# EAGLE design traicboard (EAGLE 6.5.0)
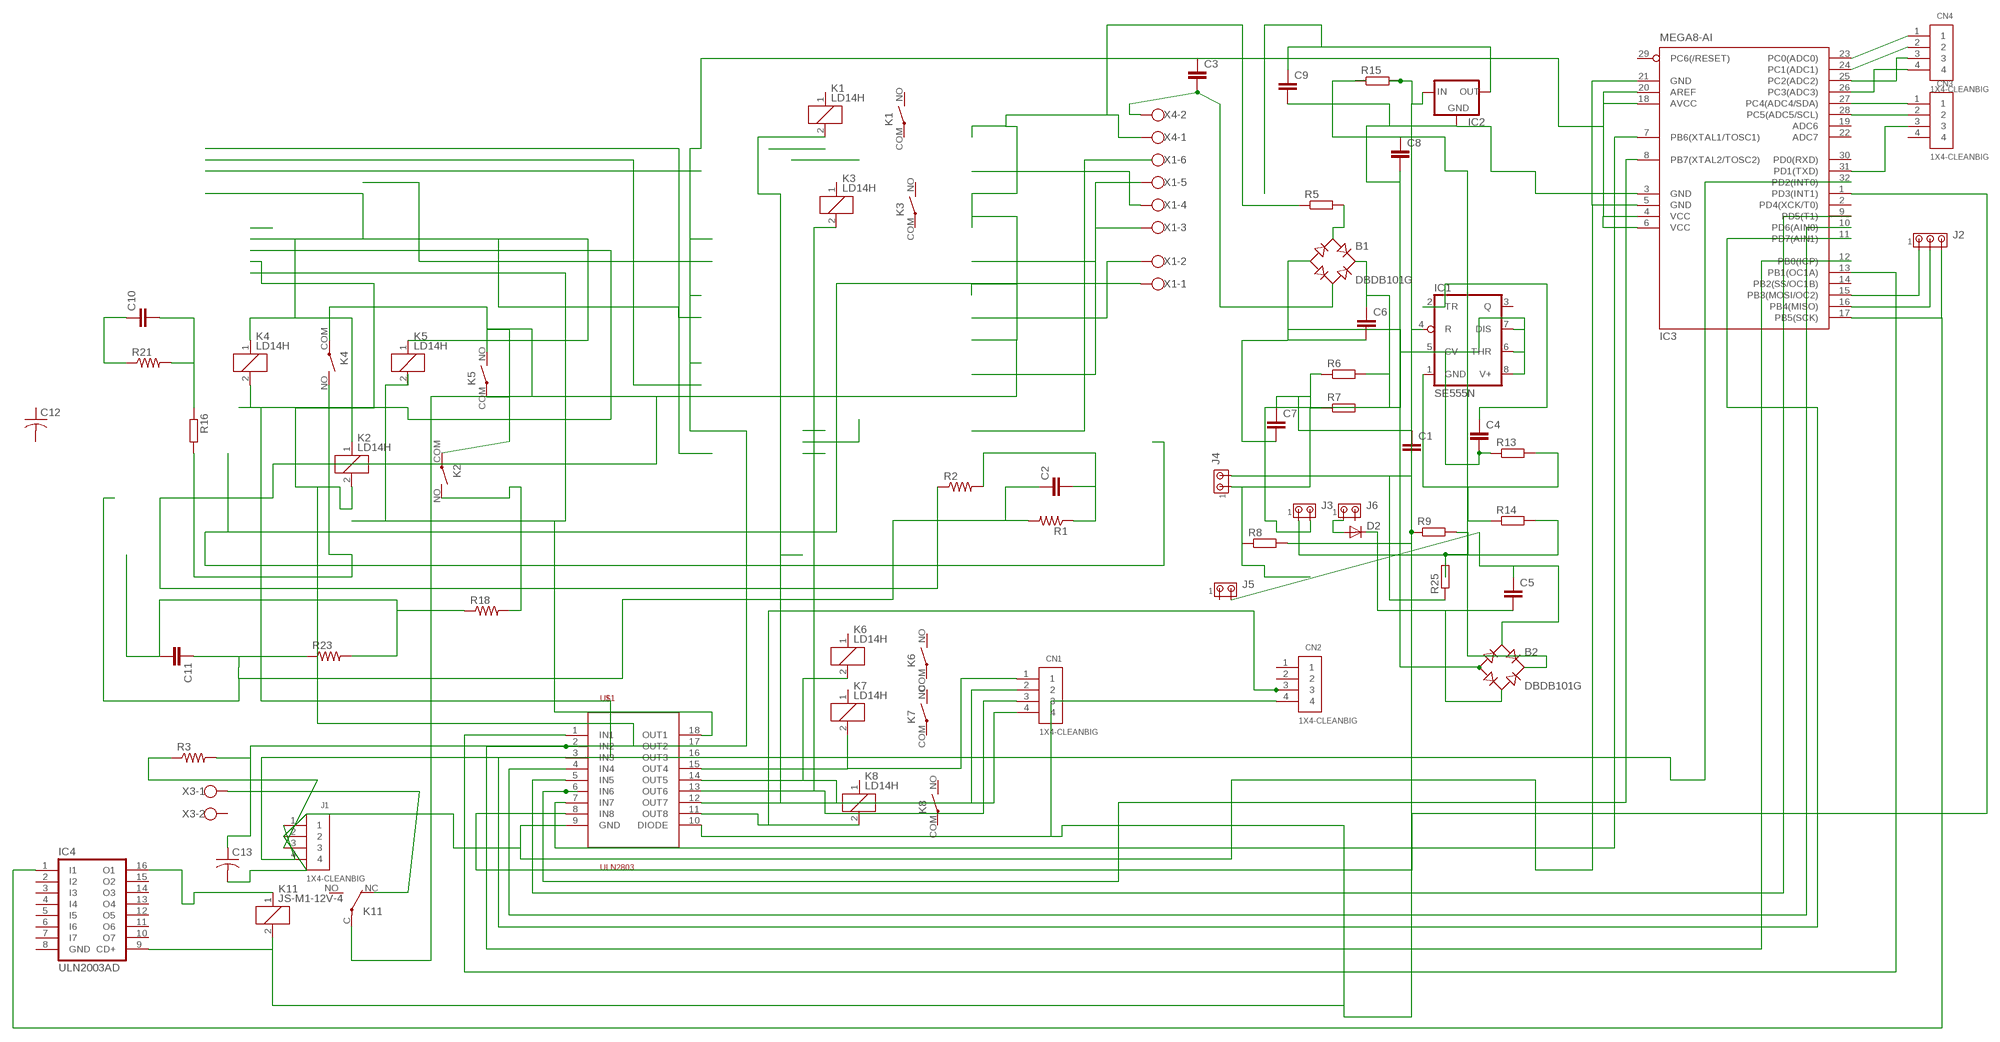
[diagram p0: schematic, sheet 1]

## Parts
B1  DBDB101G  [DB]
B2  DBDB101G  [DB]
C1  C5/2.5  [C5B2.5]
C2  C27/9  [C27.5B9]
C3  C-EU075-032X103  [C075-032X103]
C4  C-EU025-024X044  [C025-024X044]
C5  C-EU025-024X044  [C025-024X044]
C6  C5/2.5  [C5B2.5]
C7  C5/2.5  [C5B2.5]
C8  C-EU025-024X044  [C025-024X044]
C9  C-EU025-024X044  [C025-024X044]
C10  C27/9  [C27.5B9]
C11  C27/9  [C27.5B9]
C12  C-US025-024X044  [C025-024X044]
C13  C-US025-024X044  [C025-024X044]
CN1  1X4-CLEANBIG  [1X04-CLEANBIG]
CN2  1X4-CLEANBIG  [1X04-CLEANBIG]
CN3  1X4-CLEANBIG  [1X04-CLEANBIG]
CN4  1X4-CLEANBIG  [1X04-CLEANBIG]
D2  DIODE-C1702-05  [C1702-05]
IC1  SE555N  [DIL08]
IC2  V_REG_78XXSIDE  [78XXL]
IC3  MEGA8-AI  [TQFP32-08]
IC4  ULN2003AD  [SO16]
J1  1X4-CLEANBIG  [1X04-CLEANBIG]
J2  MTA03-100  [10X03MTA]
J3  MTA02-100  [10X02MTA]
J4  MTA02-100  [10X02MTA]
J5  MTA02-100  [10X02MTA]
J6  MTA02-100  [10X02MTA]
K1  LD14H  [LD]
K2  LD14H  [LD]
K3  LD14H  [LD]
K4  LD14H  [LD]
K5  LD14H  [LD]
K6  LD14H  [LD]
K7  LD14H  [LD]
K8  LD14H  [LD]
K11  JS-M1-12V-4  [JS-M]
R1  R-US_0207/15  [0207/15]
R2  R-US_0617/5V  [0617V]
R3  R-US_0204/2V  [0204V]
R5  R-EU_0414/5V  [0414V]
R6  R-EU_0204/2V  [0204V]
R7  R-EU_0204/2V  [0204V]
R8  R-EU_0204/2V  [0204V]
R9  R-EU_0204/2V  [0204V]
R13  R-EU_0204/2V  [0204V]
R14  R-EU_0204/2V  [0204V]
R15  R-EU_0414/5V  [0414V]
R16  R-EU_0411/3V  [0411V]
R18  R-US_0817/7V  [P0817V]
R21  R-US_0207/10  [0207/10]
R23  R-US_0817/22  [P0817/22]
R25  R-EU_0204/2V  [0204V]
U$1  ULN2803  [SO18L]
X1  W237-136  [W237-136]
X3  W237-102  [W237-102]
X4  W237-102  [W237-102]

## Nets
DIODE: CN2.4 IC2.IN IC4.9(CD+) K11.2 R15.2 U$1.10(DIODE)
GND: B2.- C8.2 C9.2 C13.2 IC2.GND IC3.3(GND) IC3.5(GND) IC3.21(GND) J1.2 U$1.9(GND)
N$1: K4.NO(2:S) R16.2
N$2: X1.4
N$3: X1.3
N$4: X1.2
N$6: C2.1 C11.1 R1.2 R23.1
N$7: X1.1
N$8: K2.NO(2:S) R18.2
N$10: CN1.1 K7.2 U$1.15(OUT4)
N$12: K4.2 U$1.16(OUT3)
N$13: K2.COM(2:P) K4.COM(2:P) K5.COM(2:P)
N$14: K2.2 U$1.17(OUT2)
N$15: K2.1 K4.1 K5.1
N$16: J1.3 R3.1
N$19: CN2.3 K8.2 U$1.11(OUT8)
N$20: CN1.4 K1.2 U$1.12(OUT7)
N$21: X1.6
N$23: CN1.3 K3.2 U$1.13(OUT6)
N$24: CN1.2 K6.2 U$1.14(OUT5)
N$25: IC3.1(PD3(INT1)) U$1.8(IN8)
N$27: IC3.7(PB6(XTAL1/TOSC1)) U$1.7(IN7)
N$28: IC3.8(PB7(XTAL2/TOSC2)) U$1.6(IN6)
N$29: IC3.9(PD5(T1)) U$1.5(IN5)
N$31: K11.C(2:P) R5.1 X4.1
N$33: X1.5
N$34: IC3.10(PD6(AIN0)) U$1.4(IN4)
N$35: IC3.11(PD7(AIN1)) U$1.3(IN3)
N$36: K5.NO(2:S) R2.1
N$40: B1.AC1 R5.2
N$41: B1.AC2 C3.2 X4.2
N$42: B1.- C4.2 C6.2 C7.2 IC1.5(CV) IC1.6(THR) IC1.7(DIS) IC1.8(V+) J3.2 R13.1
N$43: B1.+ C6.1 R6.2 R7.2
N$44: R9.2 R25.2
N$46: C1.2 R8.2 R9.1
N$47: C1.1 C7.1 J4.1 R6.1 R7.1 R8.1
N$48: IC1.4(R) J4.2 R25.1
N$49: IC1.1(GND) R13.2 R14.1
N$50: B2.AC1 C5.1 J5.2
N$51: C4.1 IC1.2(TR)
N$52: J3.1 R14.2
N$53: D2.A J6.1
N$54: B2.AC2 C5.2 D2.C
N$55: B2.+ C8.1 R15.1
N$56: K11.NC(2:O) X3.1
N$57: IC3.12(PB0(ICP)) U$1.2(IN2)
N$58: K5.2 U$1.18(OUT1)
N$62: C10.2 R16.1 R21.2
N$63: C10.1 R21.1
N$64: IC3.13(PB1(OC1A)) U$1.1(IN1)
N$65: C11.2 R18.1 R23.2
N$66: C2.2 R1.1 R2.2
N$68: IC3.15(PB3(MOSI/OC2)) J2.1
N$69: IC3.16(PB4(MISO)) J2.2
N$70: IC3.17(PB5(SCK)) IC4.1(I1) J2.3
N$71: IC3.32(PD2(INT0)) J1.1
N$72: C9.1 C13.1 IC2.OUT IC3.4(VCC) IC3.6(VCC) IC3.18(AVCC) IC3.20(AREF) R3.2
N$73: IC4.16(O1) K11.1
N$74: CN4.1 IC3.23(PC0(ADC0))
N$75: CN4.2 IC3.24(PC1(ADC1))
N$76: CN4.3 IC3.25(PC2(ADC2))
N$77: CN3.1 IC3.27(PC4(ADC4/SDA))
N$78: CN4.4 IC3.26(PC3(ADC3))
N$79: CN3.2 IC3.28(PC5(ADC5/SCL))
N$80: CN3.3 IC3.31(PD1(TXD))
Unconnected: C3.1 C12.1 C12.2 CN2.1 CN2.2 CN3.4 IC1.3(Q) IC3.2(PD4(XCK/T0)) IC3.14(PB2(SS/OC1B)) IC3.19(ADC6) IC3.22(ADC7) IC3.29(PC6(/RESET)) IC3.30(PD0(RXD)) IC4.2(I2) IC4.3(I3) IC4.4(I4) IC4.5(I5) IC4.6(I6) IC4.7(I7) IC4.10(O7) IC4.11(O6) IC4.12(O5) IC4.13(O4) IC4.14(O3) IC4.15(O2) J1.4 J5.1 J6.2 K1.1 K1.COM(2:P) K1.NO(2:S) K3.1 K3.COM(2:P) K3.NO(2:S) K6.1 K6.COM(2:P) K6.NO(2:S) K7.1 K7.COM(2:P) K7.NO(2:S) K8.1 K8.COM(2:P) K8.NO(2:S) K11.NO(2:S) X3.2

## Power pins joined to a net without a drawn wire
GND: IC4.8(GND)

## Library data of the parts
B1 B2 = rectifier:DB?*G: Single Phase 1.0 AMP Glass Passivated Bridge Rectifier Taiwan Semiconductor Co.,Ltd. - TSC Source: http://www.taiwansemi.com/TSCbig5/ezcatfiles/cust/img/img/db101g.pdf http://www.ts.com.tw/db/pictures/modules/PDT/PDT060207001/DBLS201G.pdf
C1 C2 C6 C7 C10 C11 = capacitor-wima:C: CAPACITOR
C3-C5 C8 C9 = rcl:C-EU: CAPACITOR, European symbol
C12 C13 = adafruit:C-US: CAPACITOR, American symbol
CN1-CN4 J1 = adafruit:1X4: 4-pin connector
D2 = diode:DIODE-: DIODE
IC1 = linear:*555: TIMER
IC2 = SparkFun-3-2-07:V_REG_78XX: Voltage Regulator Standard 7805 5V regulator. IGO (Input Ground Output). Spark Fun Electronics SKU : IC-VReg-5V
IC3 = atmel:MEGA8: MICROCONTROLLER 8 Kbytes FLASH, 1 kbytes SRAM, 512 bytes EEPROM, USART, 6-channel 10 bit ADC, 2-channel 8 bit ADC Pin compatible with Atmega48, ATMega88, ATMega168 Source: avr.lbr; MPN: ATMEGA8-16AU; OC_FARNELL: 9171371; OC_NEWARK: 73M8863
IC4 = uln-udn:ULN2003A: DRIVER ARRAY
J2 = con-amp:MTA03-100: AMP connector
J3-J6 = con-amp:MTA02-100: AMP connector
K1-K8 = relay:LD?*: Slim Power Relay NAiS Source: http://www.mew-europe.com/.. en_ds_61112_0000.pdf; OC_FARNELL: unknown; OC_NEWARK: unknown
K11 = relay:JS-M1*: Automotive Ultra-Miniature Power Relay NAiS Source: http://www.mew-europe.com/.. en_ds_61211_0000.pdf; MPN: JSM1-12V-4; OC_FARNELL: 910338; OC_NEWARK: 13P4552
R1-R3 R18 R21 R23 = adafruit:R-US_: RESISTOR, American symbol
R5-R9 R13-R16 R25 = rcl:R-EU_: RESISTOR, European symbol
U$1 = uln2803:ULN2803
X1 = con-wago-500:W237-136: WAGO SCREW CLAMP; MPN: 237-136; OC_FARNELL: unknown; OC_NEWARK: 84K9151
X3 X4 = con-wago-500:W237-102: WAGO SCREW CLAMP; MPN: 237-102; OC_FARNELL: unknown; OC_NEWARK: 70K9898

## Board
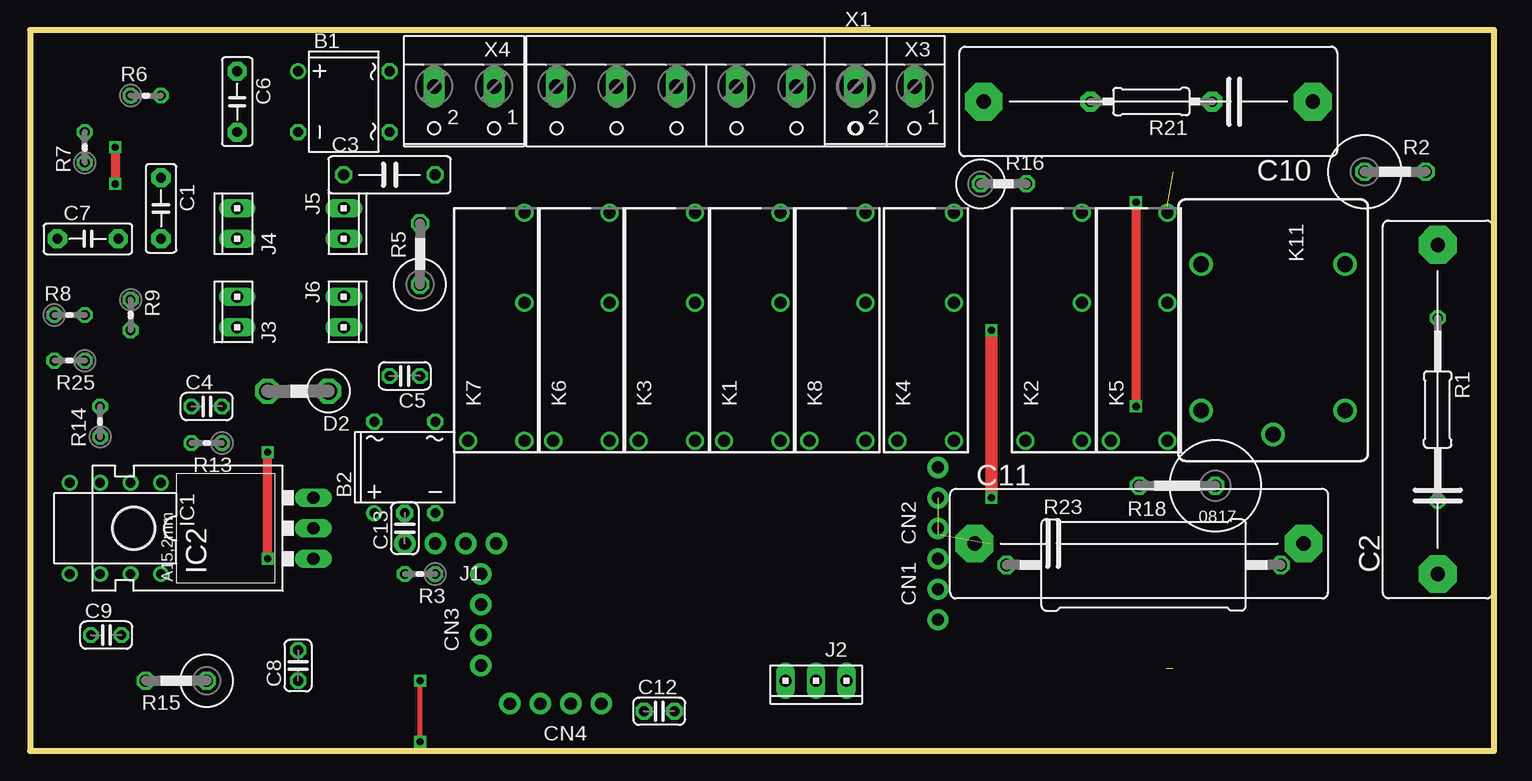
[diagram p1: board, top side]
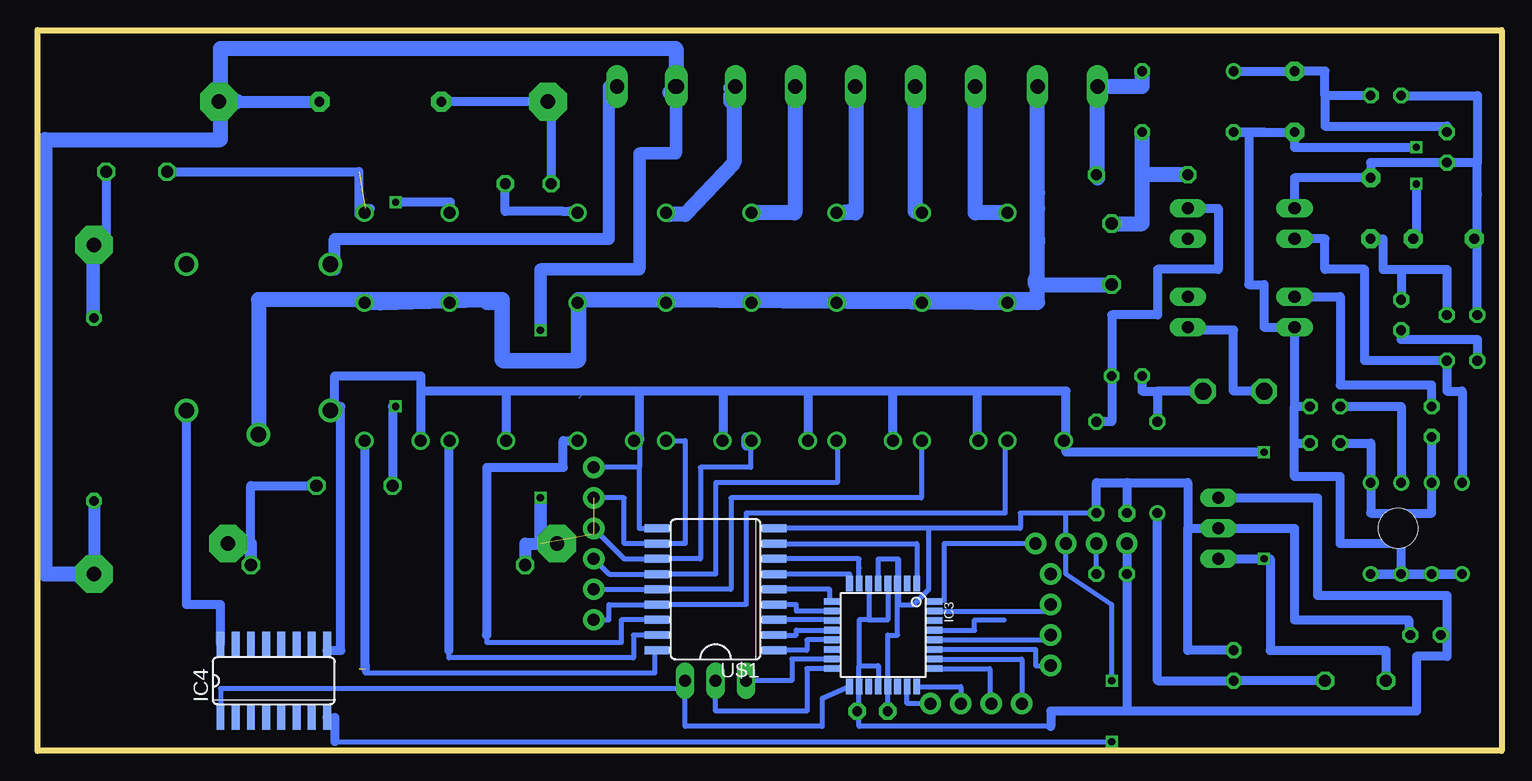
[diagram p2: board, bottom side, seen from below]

Size 122.05 x 60.07 mm. Coordinates in mm from the lower left corner, seen from the top.
Outline: 0,0 122.05,0 122.05,60.07 0,60.07 0,0
Copper layers (1*16): Top 0.035mm / dielectric 1.5mm / Bottom 0.035mm
Design rules "default": minimum track width 10mil, minimum drill 24mil, track to track 8mil, track to pad 8mil, pad to pad 8mil, via to via 8mil, smd to smd 8mil, copper to edge 40mil, drill to drill 8mil, minimum pad ring 10mil, minimum via ring 8mil, stop-mask expansion 4mil, vias tented up to drill 0mil, thermal gap 10mil

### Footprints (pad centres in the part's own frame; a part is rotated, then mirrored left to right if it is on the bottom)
DB = drill 0.813: + -2.54,-3.81 | drill 0.813 octagon: - 2.54,-3.81; AC1 2.54,3.81; AC2 -2.54,3.81
C5B2.5 = drill 0.813 pad 1.6 octagon: 1 -2.54,0; 2 2.54,0
C27.5B9 = drill 1.194 pad 3.15 octagon: 1 -13.716,0; 2 13.716,0
C075-032X103 = drill 0.914 octagon: 1 -3.81,0; 2 3.81,0
C025-024X044 = drill 0.813 octagon: 1 -1.27,0; 2 1.27,0
C025-024X044' = drill 0.813 pad 1.422 octagon: 1 -1.27,0; 2 1.27,0
1X04-CLEANBIG = drill 1.016 pad 1.778: 1 -3.81,0; 2 -1.27,0; 3 1.27,0; 4 3.81,0
C1702-05 = drill 1.397 octagon: A 2.54,0; C -2.54,0
DIL08 = drill 0.813 pad 1.27: 1 -3.81,-3.81; 2 -1.27,-3.81; 3 1.27,-3.81; 4 3.81,-3.81; 5 3.81,3.81; 6 1.27,3.81; 7 -1.27,3.81; 8 -3.81,3.81
78XXL = drill 1.016 long: GND 0,-3.81; IN -2.54,-3.81; OUT 2.54,-3.81 | hole 3.302: 0,11.176
TQFP32-08 = smd 1.27 x 0.559: 1 -4.293,2.8; 2 -4.293,2; 3 -4.293,1.2; 4 -4.293,0.4; 5 -4.293,-0.4; 6 -4.293,-1.2; 7 -4.293,-2; 8 -4.293,-2.8; 17 4.293,-2.8; 18 4.293,-2; 19 4.293,-1.2; 20 4.293,-0.4; 21 4.293,0.4; 22 4.293,1.2; 23 4.293,2; 24 4.293,2.8 | smd 0.559 x 1.27: 9 -2.8,-4.293; 10 -2,-4.293; 11 -1.2,-4.293; 12 -0.4,-4.293; 13 0.4,-4.293; 14 1.2,-4.293; 15 2,-4.293; 16 2.8,-4.293; 25 2.8,4.293; 26 2,4.293; 27 1.2,4.293; 28 0.4,4.293; 29 -0.4,4.293; 30 -1.2,4.293; 31 -2,4.293; 32 -2.8,4.293
SO16 = smd 0.66 x 2.032: 1 -4.445,-3.073; 2 -3.175,-3.073; 3 -1.905,-3.073; 4 -0.635,-3.073; 5 0.635,-3.073; 6 1.905,-3.073; 7 3.175,-3.073; 8 4.445,-3.073; 9 4.445,3.073; 10 3.175,3.073; 11 1.905,3.073; 12 0.635,3.073; 13 -0.635,3.073; 14 -1.905,3.073; 15 -3.175,3.073; 16 -4.445,3.073
10X03MTA = drill 1.016 long: 1 2.54,0; 2 0,0; 3 -2.54,0
10X02MTA = drill 1.016 long: 1 1.27,0; 2 -1.27,0
LD = drill 1: 1 -9.2,2.35; 2 -9.2,-2.35; COM 2.3,-2.35; NO 9.8,-2.35
JS-M = drill 1.3: 1 6.7,6; 2 6.7,-6; C 8.7,0; NC -5.5,-6; NO -5.5,6
0207/15 = drill 0.813 octagon: 1 -7.62,0; 2 7.62,0
0617V = drill 1.016 octagon: 1 -2.54,0; 2 2.54,0
0204V = drill 0.813 octagon: 1 -1.27,0; 2 1.27,0
0414V = drill 1.016 octagon: 1 -2.54,0; 2 2.54,0
0411V = drill 0.914 octagon: 1 -2.54,0; 2 1.27,0
P0817V = drill 1.016 octagon: 1 -5.08,0; 2 1.27,0
0207/10 = drill 0.813 pad 1.676 octagon: 1 -5.08,0; 2 5.08,0
P0817/22 = drill 1.016 octagon: 1 -11.43,0; 2 11.43,0
SO18L = smd 0.66 x 2.032: 1 -5.08,-4.902; 2 -3.81,-4.902; 3 -2.54,-4.902; 4 -1.27,-4.902; 5 0,-4.902; 6 1.27,-4.902; 7 2.54,-4.902; 8 3.81,-4.902; 9 5.08,-4.902; 10 5.08,4.902; 11 3.81,4.902; 12 2.54,4.902; 13 1.27,4.902; 14 0,4.902; 15 -1.27,4.902; 16 -2.54,4.902; 17 -3.81,4.902; 18 -5.08,4.902
W237-136 = drill 1.194 long: 1 -12.5,-1.27; 2 -7.5,-1.27; 3 -2.5,-1.27; 4 2.5,-1.27; 5 7.5,-1.27; 6 12.5,-1.27
W237-102 = drill 1.194 long: 1 -2.5,-1.27; 2 2.5,-1.27

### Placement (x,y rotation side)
B1  26.16,54.1 270 top
B2  31.24,23.62 0 top
C1  10.92,45.21 270 top
C2  117.35,28.45 90 top
C3  29.97,48.01 0 top
C4  14.73,28.7 0 top
C5  31.24,31.24 180 top
C6  17.27,54.1 270 top
C7  4.83,42.67 0 top
C8  22.35,7.11 90 top
C9  6.35,9.65 0 top
C10  93.22,54.1 180 top
C11  92.46,17.27 0 top
C12  [C025-024X044']  52.45,3.3 0 top
C13  [C025-024X044']  31.24,18.54 90 top
CN1  75.69,14.73 90 top
CN2  75.69,19.81 90 top
CN3  37.59,10.92 90 top
CN4  43.81,3.94 180 top
D2  22.35,29.97 180 top
IC1  7.11,18.54 180 top
IC2  19.81,18.54 90 top
IC3  51.56,9.65 270 bottom
IC4  102.36,5.84 0 bottom
J1  35.05,17.27 180 top
J2  65.53,5.84 180 top
J3  17.27,36.58 90 top
J4  17.27,43.94 90 top
J5  26.16,43.94 270 top
J6  26.16,36.58 270 top
K1  60.2,35.05 90 top
K2  85.34,35.05 90 top
K3  53.09,35.05 90 top
K4  74.68,35.05 90 top
K5  92.46,35.05 90 top
K6  45.97,35.05 90 top
K7  38.86,35.05 90 top
K8  67.31,35.05 90 top
K11  103.63,35.05 270 top
R1  117.35,28.45 270 top
R2  113.79,48.26 0 top
R3  32.51,14.73 180 top
R5  32.51,41.4 90 top
R6  9.65,54.61 0 top
R7  4.57,50.29 90 top
R8  3.3,36.32 0 top
R9  8.38,36.32 270 top
R13  14.73,25.65 180 top
R14  5.84,27.43 90 top
R15  12.19,5.84 180 top
R16  81.79,47.24 0 top
R18  93.73,22.1 180 top
R21  93.47,54.1 180 top
R23  92.84,15.49 0 top
R25  3.3,32.51 180 top
U$1  65.53,13.46 90 bottom
X1  56.39,54.1 180 top
X3  71.25,54.1 180 top
X4  36.2,54.1 180 top

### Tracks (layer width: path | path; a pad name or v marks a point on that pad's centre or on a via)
DIODE  (via drill 0.6)  (1 unrouted)
  Top 0.762: v19.81,16 v19.81,24.89
  Bottom 0.406: 36.32,29.97 71.88,29.97 | U$1.10 71.88,18.54 71.88,23.62 | K11.2 97.28,28.35 | IC4.9 97.92,8.38 | 96.77,8.38 96.65,13.46 | 71.88,29.97 71.88,23.62 | 71.88,29.97 90.11,29.97 | 71.88,23.62 CN2.4
  Bottom 0.762: R15.2 9.65,8.38 19.3,8.38 19.3,16 v19.81,16 IC2.IN | v19.81,24.89 36.32,24.89 36.32,29.97 | 97.28,28.7 97.28,31.24 90.11,31.24 90.11,29.97 | 97.92,8.38 96.77,8.38 96.77,28.7 97.28,28.7 | 97.28,28.7 97.28,28.35
GND  (via drill 0.6)
  Top 0.406: v32.51,0.76 v32.51,5.84
  Bottom 0.406: IC3.21 51.18,5.36 51.18,9.65 50.36,9.65 50.36,12.26 | IC3.5 51.96,16 50.36,16 | 50.36,16 IC3.3 50.36,12.26 | B2.- 36.32,19.81 | 50.29,12.26 50.36,12.26 | 50.36,16 50.29,16 50.29,12.26 | 50.29,12.26 50.29,12.19 49.02,12.19 47.75,13.46 47.75,18.54 | 36.32,19.81 40.13,19.81 40.13,18.54 47.75,18.54 | 47.75,18.54 U$1.9 | 36.32,19.81 J1.2 36.32,14.73 32.51,12.19 v32.51,5.84 | 33.78,22.35 31.24,22.35 | 97.28,0.76 v32.51,0.76 | 47.37,10.03 43.94,10.03 43.94,10.92 41.47,10.92
  Bottom 0.762: 26.16,18.54 26.16,22.35 33.78,22.35 B2.- | 26.16,18.54 IC2.GND 17.27,18.54 17.27,10.92 7.75,10.92 7.75,9.65 C9.2 | C8.2 26.16,8.38 26.16,18.54 | 31.24,22.35 C13.2 | IC4.8 97.28,2.77 97.28,0.76
N$1
  Bottom 0: 80.77,44.85 K4.NO 78.23,44.96
  Bottom 0.762: K4.NO 77.22,44.96 77.72,44.96 78.23,44.96 83.06,44.96 R16.2
N$2
  Bottom 0: 53.85,44.83 54.1,47.75
  Bottom 0.254: 54.1,55.37 X1.4 53.85,55.37
  Bottom 1.27: 53.85,55.37 53.85,44.83 55.12,44.83 54.1,44.96
N$3
  Bottom 0.254: X1.3 58.93,55.37
  Bottom 1.27: 59,55.37 58.93,55.37 58.93,44.83 62.23,44.83
N$4
  Bottom 0.254: X1.2
  Bottom 1.27: X1.2 63.88,55.25 64.26,55.25 64.01,55.37 64.01,49.02 68.07,44.7 69.34,44.7
N$5
  Bottom 0.762: 36.45,29.97 43.69,29.97 | 43.69,26.16 43.69,29.97 | 43.69,29.97 50.72,29.97 | 50.72,26.16 50.72,29.97 | 50.72,29.97 57.78,29.97 | 57.78,26.16 57.78,29.97 | 57.78,29.97 64.9,29.97 | 64.9,29.97 64.9,26.16 | 64.9,29.97 83.31,29.97
N$6  (via drill 0.6)
  Top 1.016: v80.14,35.05 v80.14,21.08
  Bottom 1.016: R1.2 C2.1 | R23.1 81.41,17.27 80.14,17.27 | 68.83,58.55 68.83,49.78 71.88,49.78 71.88,40.13 80.14,40.13 v80.14,35.05 | v80.14,21.08 80.14,17.27 | 80.14,17.27 C11.1
  Bottom 1.27: C2.1 121.41,14.73 121.41,50.93 106.81,50.93 106.81,58.55 68.83,58.55
N$7
  Bottom 1.27: 105.41,54.1 106.81,54.1 106.81,58.55 68.83,58.55 68.83,55.37 | 69.34,54.86 68.83,55.37 | 68.83,55.37 X1.1
N$8  (via drill 0.6)
  Top 0.762: v92.2,45.72 v92.2,28.7
  Bottom 0.762: K2.NO 87.63,44.85 87.63,45.72 v92.2,45.72 | v92.2,28.7 92.46,28.7 R18.2
N$10
  Bottom 0.406: K7.2 41.4,25.85 41.4,19.81 62.99,19.81 62.99,12.19 U$1.15 | U$1.15 70.61,12.19 | CN1.1 74.42,10.92 74.42,12.19 U$1.15
N$11
  Bottom 0.762: 62.99,25.4 62.99,26.16 62.53,26.16 62.53,25.65
N$12
  Bottom 0.406: U$1.16 73.41,10.92 73.41,9.02 84.58,9.02 84.58,9.65
  Bottom 0.762: 84.65,9.65 84.58,9.65 84.58,23.62 78.23,23.62 78.23,25.85 K4.2
N$13
  Bottom 0: 38.68,42.67 38.86,41.16 38.68,37.35 38.86,38.86 37.59,38.66 36.58,38.66
  Bottom 0.762: 93.47,37.34 K2.COM
  Bottom 1.27: 83.31,37.59 84.58,37.35 83.31,37.35 83.31,32.51 | 83.31,37.59 83.31,32.51 | 83.31,32.51 76.96,32.51 | 76.96,32.51 76.96,37.35 | 76.96,37.35 K4.COM 76.96,37.35 | 92.2,37.35 93.47,37.34 | 92.2,37.35 K5.COM | 76.96,37.35 76.96,32.51 | 76.96,32.51 83.31,32.51 | 83.31,32.51 83.31,37.59 | 83.31,37.59 92.2,37.35 | 83.31,32.51 76.96,32.51 | 76.96,32.51 76.96,37.35 | 76.96,37.35 76.96,37.59 70.61,37.59 38.68,37.35 38.68,42.67
N$14
  Bottom 0.406: U$1.17 72.39,9.65 72.39,7.75 87.76,7.75 87.76,8.38
  Bottom 0.762: 87.76,8.38 87.76,26.16 K2.2
N$15
  Bottom 0: 76.45,29.97 71.88,29.97
  Bottom 0.025: 76.45,29.97 76.96,29.34
  Bottom 0.762: K4.1 71.88,25.85 71.88,25.91 71.88,26.16 71.88,29.97 82.99,29.97 | 82.99,29.97 K2.1 | 82.99,29.97 90.11,29.97 K5.1
N$16
  Bottom 0.406: R3.1 J1.3
N$19
  Bottom 0.406: K8.2 68.07,25.85 68.07,17.27 U$1.11 73.15,17.27 73.15,21.08 CN2.3
N$20
  Bottom 0.406: K1.2 62.61,26.16 62.61,23.62 66.8,23.62 66.8,16 U$1.12 73.15,16 CN1.4
N$21
  Bottom 1.27: 41.35,44.83 43.89,44.83 X1.6
N$23
  Bottom 0.406: K3.2 55.37,25.85 55.37,22.35 65.53,22.35 65.53,14.73 U$1.13 74.42,14.73 CN1.3
N$24
  Bottom 0.406: K6.2 48.39,25.85 48.39,21.08 64.26,21.08 64.26,13.46 U$1.14 CN1.2
N$25
  Bottom 0.406: U$1.8 48.76,17.27 IC3.1
N$27
  Bottom 0.406: U$1.7 53.58,16 53.58,15.23 IC3.7 | 51.18,3.3 51.18,5.84
N$28
  Bottom 0.406: IC3.8 54.36,14.73 U$1.6
N$29
  Bottom 0.406: IC3.9 56.01,12.45 56.01,13.46 U$1.5
N$31
  Bottom 0: 38.68,42.42 38.86,41.15 38.86,42.67
  Bottom 0.254: X4.1 | 38.68,45.21 38.86,42.67 38.8,38.86 38.86,40.13 38.86,41.15 | 38.86,47.75 38.68,46.48
  Bottom 0.406: 38.8,38.86 38.86,38.86 38.86,37.59
  Bottom 1.27: 38.68,42.42 38.68,45.21 38.68,46.48 X4.1 | 38.8,38.86 R5.1 | 38.86,37.59 76.96,37.59 76.96,32.51 83.31,32.51 83.31,37.59 103.63,37.59 K11.C
N$33
  Bottom 1.27: 48.26,44.96 48.89,44.96 X1.5
N$34
  Bottom 0.406: IC3.10 58.8,11.65 58.8,12.19 U$1.4
N$35
  Bottom 0.406: IC3.11 55.92,10.92 U$1.3
N$36  (1 unrouted)
  Bottom 0.762: 95.25,44.83 94.74,44.83 94.74,45.21 | 94.74,45.21 K5.NO 94.3,45.21 94.74,45.21 | 95.25,44.83 95.25,48.26 R2.1 | 94.74,45.21 95.25,44.7 95.25,44.83
N$37
  Bottom 1.27: 38.86,38.86 38.86,39.37
N$38
  Bottom 1.27: 38.86,55.37 38.86,55.88
N$39  (1 unrouted)
N$40
  Bottom 1.27: R5.2 29.97,43.94 29.97,48.01 | 29.97,48.01 B1.AC1 | 26.16,48.01 29.97,48.01
N$41
  Bottom 1.27: B1.AC2 29.97,55.37 X4.2 33.7,47.75 C3.2
N$42  (via drill 0.6)
  Top 0.762: v7.11,50.29 v7.11,47.24
  Bottom 0: IC1.8 10.92,15.24
  Bottom 0.762: B1.- C6.2 17.27,50.29 v7.11,50.29 | v7.11,47.24 7.11,42.67 C7.2 | IC1.7 8.38,17.27 13.46,17.27 13.46,22.86 17.27,22.86 17.27,25.65 | IC1.7 IC1.8 IC1.5 IC1.6 IC1.7 | 17.27,28.7 J3.2 19.81,35.31 19.81,38.86 21.08,38.86 21.08,51.56 B1.- | 19.81,51.56 B1.- | 17.27,25.65 R13.1 | 17.27,28.7 C4.2 | 17.27,25.65 17.27,28.7
N$43
  Bottom 0.762: 14.73,54.61 14.73,52.07 4.57,52.07 R7.2 | B1.+ C6.1 14.73,56.64 14.73,54.61 | R6.2 14.73,54.61
N$44
  Bottom 0.762: R9.2 8.38,34.29 2.03,34.29 R25.2
N$45
  Bottom 1.27: 64.26,54.1 64.26,54.61
N$46
  Bottom 0.762: 8.38,40.13 4.57,40.13 R8.2 | C1.2 9.91,42.67 9.91,40.13 8.38,40.13 | 8.38,40.13 R9.1
N$47
  Bottom 0.762: 2.03,49.02 2.02,46.36 2.03,46.36 | R8.1 2.03,42.67 | J4.1 17.27,47.75 C1.1 10.92,49.02 R7.1 2.03,49.02 | R6.1 2.03,54.61 2.03,49.02 | 2.03,46.36 2.03,49.02 | C7.1 2.03,42.67 | 2.03,42.67 2.03,46.36
N$48
  Bottom 0.762: J4.2 14.73,42.67 14.73,40.13 11.43,40.13 11.43,32.51 R25.1 4.57,29.97 3.3,29.97 IC1.4
N$49
  Bottom 0.762: R13.2 10.92,25.65 IC1.1 10.92,19.81 5.84,19.81 R14.1
N$50
  Bottom 0.762: J5.2 23.62,45.21 23.62,40.13 28.7,40.13 28.7,36.32 32.51,36.32 C5.1 32.51,27.43 B2.AC1
N$51
  Bottom 0.762: C4.1 8.38,28.7 IC1.2
N$52
  Bottom 0.762: J3.1 13.46,37.85 13.46,30.48 5.84,30.48 R14.2
N$53
  Bottom 0.762: D2.A 22.35,29.97 22.35,35.05 26.16,35.05 J6.1
N$54
  Bottom 0.762: D2.C 28.7,29.97 | C5.2 29.97,29.97 28.7,29.97 | 28.7,29.97 B2.AC2
N$55
  Bottom 0.762: B2.+ 28.7,5.84 C8.1 R15.1
N$56
  Bottom 0.406: K11.NC 97.28,40.55
  Bottom 1.016: 97.28,40.13 97.28,40.55 97.28,42.67 74.42,42.67 74.42,55.37 X3.1
N$57
  Bottom 0.406: U$1.2 58.8,9.65 58.8,10.05 IC3.12
N$58  (1 unrouted)
  Bottom 0: 69.85,8.64 70.61,8.64 70.61,6.48
  Bottom 0.406: 94.74,7.11 94.74,6.48 70.61,6.48 70.61,8.38 U$1.18
  Bottom 0.762: 94.74,6.86 94.74,7.11 94.74,25.85 K5.2
N$62
  Bottom 0: 79.5,47.75 R16.1
  Bottom 0.762: R16.1 79.25,54.1 C10.2 R21.2
N$63
  Bottom 1.016: C10.1 R21.1
N$64
  Bottom 0.406: IC3.13 57.91,9.25 57.91,8.38 U$1.1
N$65
  Bottom 0: 105.41,18.03 106.43,17.53 106.17,17.53 106.17,16.76
  Bottom 0.762: C11.2 106.17,16.76 106.43,16.76 | 105.41,18.03 106.43,16.76 | 106.43,16.76 104.27,17.27 104.27,22.1 R18.1
  Bottom 1.016: C11.2 104.27,17.27 R23.2
N$66
  Bottom 0.762: R2.2 116.33,42.67 | 116.33,42.67 116.33,42.42 117.6,42.42 | 116.33,42.67 117.6,42.67 117.6,36.32 R1.1
  Bottom 1.016: R1.1 C2.2
N$67  (via drill 0.6)  (2 unrouted)
  Top 1.016: v80.14,21.08 v80.14,35.05
  Bottom 1.016: v80.14,35.05 80.14,40.13 71.88,40.13 71.88,49.78 68.83,49.78 68.83,55.37 | 80.14,17.27 v80.14,21.08
N$68
  Bottom 0.406: IC3.15 59.18,7.65 59.18,5.84 J2.1
N$69
  Bottom 0.406: IC3.16 57.91,6.85 57.91,3.3 65.53,3.3 J2.2
N$70
  Bottom 0.406: IC3.17 56.64,4.35 56.64,2.03 68.07,2.03 68.07,5.21 | 68.07,5.21 106.81,5.21 IC4.1 | 68.07,5.21 J2.3
N$71
  Bottom 0.406: J1.1 46.48,17.27 46.48,12.51 47.27,12.51 IC3.32
N$72
  Bottom 0.406: IC3.6 52.76,10.92 | IC3.4 51.16,10.92 52.76,10.92 | 52.76,10.92 53.56,10.92 53.56,7.11 | 53.56,7.11 IC3.18 53.56,2.03 37.59,2.03 | 53.56,7.11 51.96,7.11 IC3.20
  Bottom 0.762: IC2.OUT 15.37,21.08 15.37,12.95 4.57,12.95 4.57,9.65 | C9.1 4.57,9.65 | 4.57,9.65 4.57,7.87 7.11,7.87 7.11,3.3 31.24,3.3 | 31.24,3.3 37.59,3.3 37.59,2.03 | C13.1 R3.2 31.24,3.3
N$73
  Bottom 0.762: IC4.16 106.81,12.19 109.63,12.19 K11.1
N$74
  Bottom 0.406: CN4.1 49.56,3.94 IC3.23
N$75
  Bottom 0.406: IC3.24 45.09,5.36 CN4.2
N$76
  Bottom 0.406: IC3.25 42.67,6.85 42.67,4.57 CN4.3
N$77
  Bottom 0.406: IC3.27 38.86,8.45 38.86,7.11 CN3.1
N$78
  Bottom 0.406: IC3.26 40,7.65 CN4.4
N$79
  Bottom 0.406: IC3.28 37.59,9.25 CN3.2
N$80
  Bottom 0.406: IC3.31 37.59,11.65 CN3.3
